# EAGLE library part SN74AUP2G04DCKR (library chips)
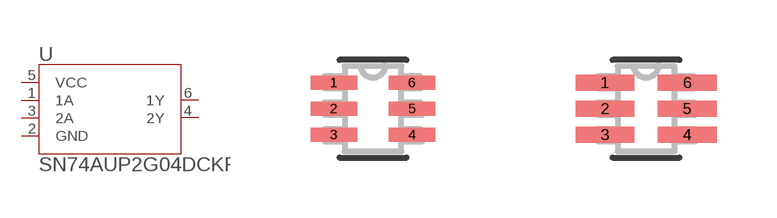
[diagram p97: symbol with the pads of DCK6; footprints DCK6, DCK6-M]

Designator prefix U

## SN74AUP2G04DCKR (MANUFACTURER_PART_NUMBER: SN74AUP2G04DCKR; VENDOR: Texas Instruments)  [DCK6]
1  1A  in
2  GND  pwr
3  2A  in
4  2Y  out
5  VCC  pwr
6  1Y  out

## SN74AUP2G04DCKRDCK6-M (MANUFACTURER_PART_NUMBER: SN74AUP2G04DCKR; VENDOR: Texas Instruments)  [DCK6-M]
Pads as for DCK6

## SN74AUP2G04DCKRDCK6-L (MANUFACTURER_PART_NUMBER: SN74AUP2G04DCKR; VENDOR: Texas Instruments)  [DCK6-L]
Pads as for DCK6

## Footprint DCK6 (pad centres in mm)
smd 1.168 x 0.356: 1 -0.978,0.65; 2 -0.978,0; 3 -0.978,-0.65; 4 0.978,-0.65; 5 0.978,0; 6 0.978,0.65

## Footprint DCK6-M (pad centres in mm)
smd 1.473 x 0.406: 1 -1.029,0.65; 2 -1.029,0; 3 -1.029,-0.65; 4 1.029,-0.65; 5 1.029,0; 6 1.029,0.65

## Footprint DCK6-L (pad centres in mm)
smd 0.864 x 0.305: 1 -0.927,0.65; 2 -0.927,0; 3 -0.927,-0.65; 4 0.927,-0.65; 5 0.927,0; 6 0.927,0.65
